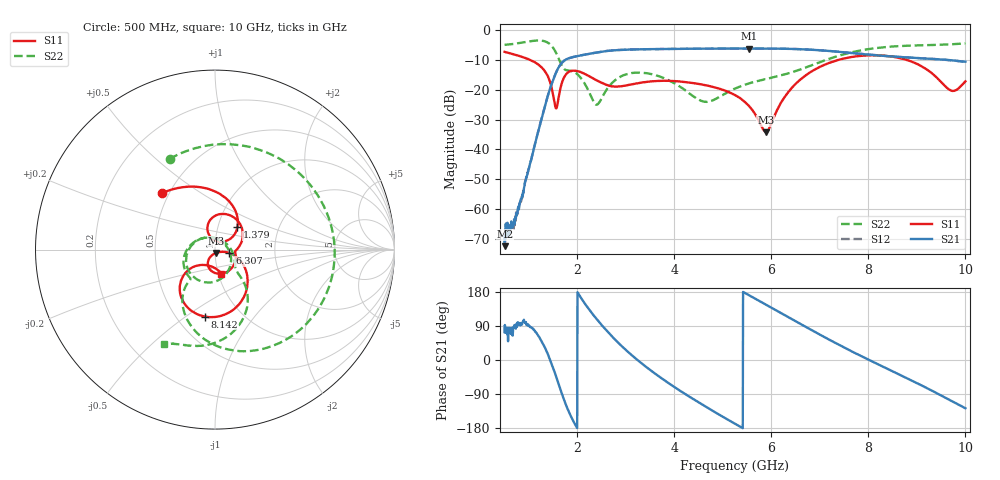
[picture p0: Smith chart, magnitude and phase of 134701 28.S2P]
!  2-Port S-parameters saved by WinCal
! VAR MeasName=S-Parameters (CALIBRATED_DATA) read from VNA (N5242A)
! VAR MeasDate=2013-7-3 16:32:54
! VAR NAME=134701 28
! VAR FILENAME=134701 28.S2P
! VAR DATE=2013-7-3 16:32:54
! VAR PHYS_PORTS=1,2
# Hz S MA R 50
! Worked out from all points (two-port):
!   1601 points, 500 MHz to 10 GHz, reference 50 ohm
!   highest |S21| = -6.20 dB at 5.535 GHz (marker M1); lowest = -72.4 dB at 505.9 MHz (marker M2)
!   |S21| within 3 dB of the highest: 1.87 GHz to 8.822 GHz (6.952 GHz wide, 130 % of centre)
!   lowest |S11| = -34.2 dB at 5.885 GHz (marker M3), VSWR 1.04, Z = 50.6 - j1.88 ohm
!   |S11| at or under -10 dB: 1.027 GHz to 7.383 GHz (6.357 GHz wide, 151 % of centre); 8.786 GHz to end of sweep
!   |S22| runs from -25.0 to -3.5 dB; largest |S21 - S12| = 0.0027
!   S11 on the Smith chart (normalised r, x): 500 MHz: 0.46, +0.36; 1.379 GHz: 1.24, +0.32; 6.307 GHz: 1.17, -0.05; 8.142 GHz: 0.68, -0.59; 10 GHz: 1.04, -0.28
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5e8  0.4308 133.0  0.0003473 73.6  0.0003532 64.5  0.5644 116.6
5.059375e8  0.4293 132.5  0.0002403 92.5  0.0002834 90.7  0.565 115.7
7.196875e8  0.3848 114.7  0.0007315 85.8  0.0007563 95.9  0.591 83.7
1.099688e9  0.2959 79.2  0.009979 80.7  0.0101 80.8  0.6609 11.2
1.37875e9  0.1762 45.0  0.07321 19.7  0.07329 19.6  0.6219 -60.5
1.562812e9  0.04876 75.3  0.1958 -43.6  0.1957 -43.7  0.412 -112.8
1.770625e9  0.1832 92.5  0.3234 -120.3  0.323 -120.3  0.2129 -129.9
2.085312e9  0.1954 41.5  0.3779 162.0  0.3779 162.0  0.1524 178.0
2.388125e9  0.1448 11.8  0.4188 109.3  0.419 109.3  0.05645 64.4
2.649375e9  0.1171 -1.7  0.4491 71.0  0.4499 71.0  0.1134 -38.3
3.130312e9  0.1237 -20.4  0.4729 11.8  0.4729 11.7  0.1908 -108.1
3.670625e9  0.1407 -53.9  0.4805 -42.2  0.4799 -42.2  0.1696 -161.7
4.620625e9  0.1201 -100.1  0.4878 -121.2  0.4878 -121.3  0.06327 73.8
5.25e9  0.08144 -119.2  0.4893 -168.3  0.4895 -168.3  0.1046 -13.9
5.535e9  0.05386 -123.2  0.49 171.2  0.4899 171.2  0.1276 -30.3
5.885312e9  0.01952 -72.2  0.4888 146.3  0.489 146.2  0.1509 -41.0
6.306875e9  0.08269 -13.5  0.4851 116.3  0.4853 116.2  0.1841 -45.8
6.835312e9  0.204 -33.2  0.4673 78.5  0.4678 78.5  0.2579 -49.7
8.141562e9  0.3774 -98.6  0.3785 -7.8  0.3798 -8.0  0.4967 -83.8
8.420625e9  0.3648 -111.6  0.3639 -25.0  0.3637 -25.3  0.5235 -91.4
9.709062e9  0.0965 -113.5  0.3116 -107.7  0.3104 -107.8  0.5782 -114.9
1e10  0.1382 -74.9  0.2947 -127.3  0.2936 -127.5  0.5963 -118.4
